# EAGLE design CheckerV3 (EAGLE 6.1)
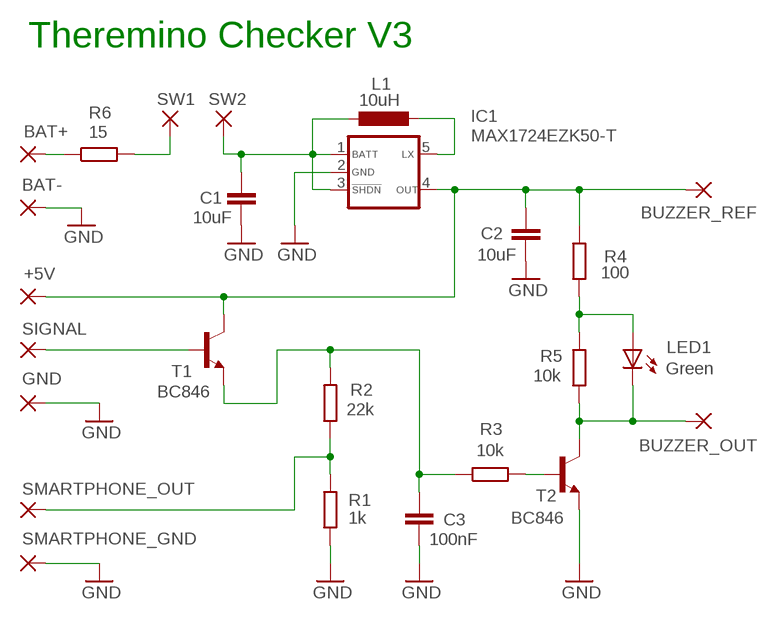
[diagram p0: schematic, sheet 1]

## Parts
+5V  WIREPADSMD1,27-254  [SMD1,27-2,54]
BAT+  WIREPAD2,54/0,9  [2,54/0,9]
BAT-  WIREPAD2,54/0,9  [2,54/0,9]
BUZZER_OUT  WIREPADSMD1,27-254  [SMD1,27-2,54]
BUZZER_REF  WIREPADSMD1,27-254  [SMD1,27-2,54]
C1  10uF  C-EUC0805  [C0805]
C2  10uF  C-EUC0805  [C0805]
C3  100nF  C-EUC0805  [C0805]
GND  WIREPADSMD1,27-254  [SMD1,27-2,54]
IC1  MAX1724EZK50-T  MAX1724SOT23-5-L08  [SOT23-5-L08]
L1  10uH  INDUCTORL1812  [L1812]
LED1  Green  LEDLED3MM-SMD  [LED3MM-SMD]
R1  1k  R-EU_R0805  [R0805]
R2  22k  R-EU_R0805  [R0805]
R3  10k  R-EU_R0805  [R0805]
R4  100  R-EU_R0805  [R0805]
R5  10k  R-EU_R0805  [R0805]
R6  15  R-EU_R0805  [R0805]
SIGNAL  WIREPADSMD1,27-254  [SMD1,27-2,54]
SMARTPHONE_GND  WIREPADSMD1,27-254  [SMD1,27-2,54]
SMARTPHONE_OUT  WIREPADSMD1,27-254  [SMD1,27-2,54]
SW1  WIREPADSMD1,27-254  [SMD1,27-2,54]
SW2  WIREPADSMD1,27-254  [SMD1,27-2,54]
T1  BC846  BC846N  [SOT23]
T2  BC846  BC846N  [SOT23]

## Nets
+BAT: C1.1 IC1.1 IC1.3 L1.1 SW2.1(P)
GND: BAT-.1(P) C1.2 C2.2 C3.2 GND.1(P) IC1.2 R1.1 SMARTPHONE_GND.1(P) T2.2(E)
N$1: LED1.A R4.2 R5.1
N$2: IC1.5 L1.2
N$3: +5V.1(P) BUZZER_REF.1(P) C2.1 IC1.4 R4.1 T1.3(C)
N$4: BUZZER_OUT.1(P) LED1.K(C) R5.2 T2.3(C)
N$5: SIGNAL.1(P) T1.1(B)
N$6: R3.2 T2.1(B)
N$7: R6.2 SW1.1(P)
N$8: C3.1 R2.2 R3.1 T1.2(E)
N$9: R1.2 R2.1 SMARTPHONE_OUT.1(P)
N$10: BAT+.1(P) R6.1

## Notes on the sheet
- Theremino Checker V3

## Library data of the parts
+5V BAT+ BAT- BUZZER_OUT BUZZER_REF GND SIGNAL SMARTPHONE_GND SMARTPHONE_OUT SW1 SW2 = wirepad:WIREPAD: Wire PAD connect wire on PCB
C1-C3 = 00-LIVIO:C-EU: CAPACITOR, European symbol
IC1 = 00-LIVIO:MAX1724: 1.5uA Step-Up DC-DC Converter
L1 = 00-LIVIO:INDUCTOR
LED1 = 00-LIVIO:LED: LEDS
R1-R6 = 00-LIVIO:R-EU_: RESISTOR, European symbol
T1 T2 = 00-LIVIO:BC846

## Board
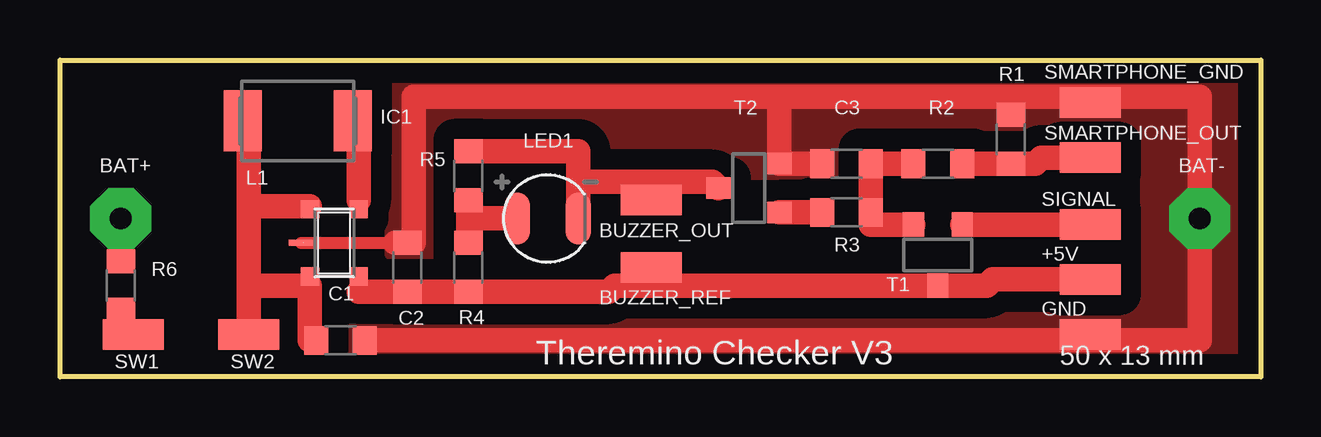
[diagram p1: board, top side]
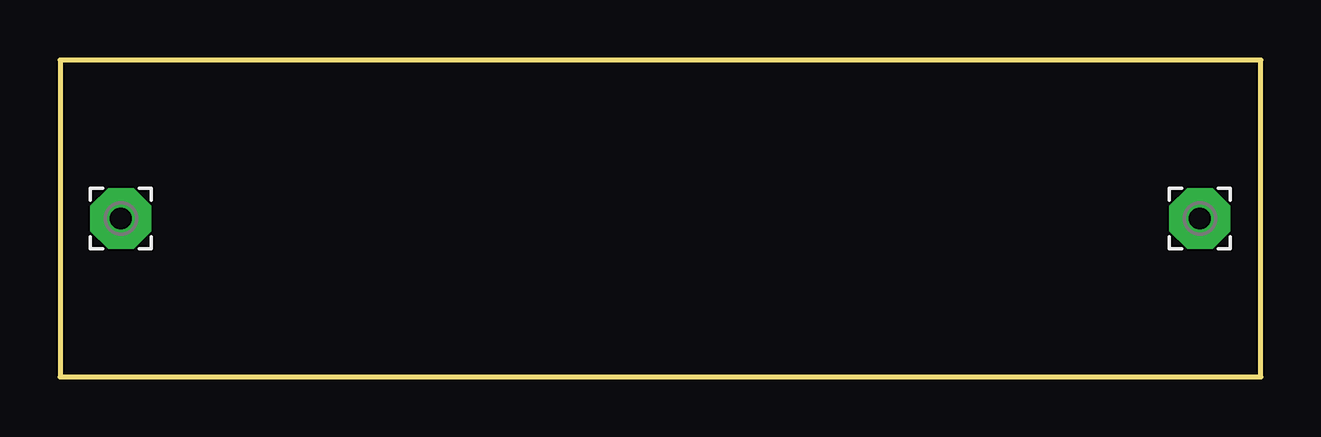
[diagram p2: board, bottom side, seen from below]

Size 50.04 x 13.21 mm. Coordinates in mm from the lower left corner, seen from the top.
Outline: 0,0 0,13.21 50.04,13.21 50.04,0 0,0
Copper layers (1*16): Top 0.035mm / dielectric 1.5mm / Bottom 0.035mm
Design rules: minimum track width 10mil, minimum drill 29mil, track to track 29mil, track to pad 29mil, pad to pad 29mil, via to via 29mil, smd to smd 29mil, copper to edge 29mil, drill to drill 8mil, minimum pad ring 5mil, minimum via ring 8mil, stop-mask expansion 4mil, vias tented up to drill 0mil, thermal gap 44mil

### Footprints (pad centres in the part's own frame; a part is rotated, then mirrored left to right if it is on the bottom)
SMD1,27-2,54 = smd 1.27 x 2.54: 1 0,0
2,54/0,9 = drill 0.914 pad 2.54 octagon: 1 0,0
C0805 = smd 1 x 1.2: 1 -1.016,0; 2 1.016,0
SOT23-5-L08 = smd 0.762 x 0.762: 1 -1.397,-1.016; 3 1.397,-1.016; 4 1.397,1.016; 5 -1.397,1.016 | smd 0.254 x 0.991: 2 0,-1.397
L1812 = smd 1.575 x 2.54: 1 -2.286,0; 2 2.286,0
LED3MM-SMD = smd 1.067 x 2.184: A -1.27,0; K 1.27,0
R0805 = smd 1 x 1.2: 1 -1.016,0; 2 1.016,0
SOT23 = smd 0.889 x 1.016: 1 -1.016,-1.27; 2 1.016,-1.27; 3 0,1.27

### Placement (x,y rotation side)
+5V  42.93,4.06 90 top
BAT+  2.54,6.6 0 bottom
BAT-  47.5,6.6 0 bottom
BUZZER_OUT  24.64,7.37 90 top
BUZZER_REF  24.64,4.57 90 top
C1  11.68,1.52 0 top
C2  14.48,4.57 90 top
C3  32.77,8.89 180 top
GND  42.93,1.78 90 top
IC1  11.43,5.59 270 top
L1  9.91,10.67 0 top
LED1  20.32,6.6 0 top
R1  39.62,9.91 270 top
R2  36.58,8.89 180 top
R3  32.77,6.86 180 top
R4  17.02,4.57 90 top
R5  17.02,8.38 90 top
R6  2.54,3.81 270 top
SIGNAL  42.93,6.35 90 top
SMARTPHONE_GND  42.93,11.43 90 top
SMARTPHONE_OUT  42.93,9.14 90 top
SW1  3.05,1.78 90 top
SW2  7.87,1.78 90 top
T1  36.58,5.08 180 top
T2  28.7,7.87 90 top

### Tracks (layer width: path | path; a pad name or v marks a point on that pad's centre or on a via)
+BAT
  Top 0.61: IC1.3 10.41,3.81 | IC1.1 10.41,7.11 | 7.87,10.67 L1.1
  Top 1.016: 10.41,7.11 7.87,7.11 | L1.1 7.87,10.67 7.87,7.11 | C1.1 10.41,1.52 10.41,3.81 7.87,3.81 | 7.87,3.81 SW2.1 | 7.87,7.11 7.87,3.81
GND
  Top 0.5: IC1.2 13.97,5.59
  Top 0.61: 14.73,5.59 14.73,11.68
  Top 1.016: C3.2 T2.2 29.97,11.68 | 13.97,5.59 C2.2 | C2.2 14.73,5.59 | 43.18,1.52 47.5,1.52 BAT-.1 47.5,11.68 42.93,11.68 | 43.18,1.52 42.93,1.52 GND.1 | 14.73,5.59 14.73,11.68 29.97,11.68 | 29.97,11.68 39.62,11.68 | R1.1 39.62,11.68 | SMARTPHONE_GND.1 42.93,11.68 | C1.2 40.39,1.52 43.18,1.52 | 42.93,11.68 39.62,11.68 | C2.2 14.73,5.59
  pour Top (isolate 0.85, rank 6, no thermals): -1,-1 51.04,-1 51.04,14.21 -1,14.21
N$1
  Top 1.016: LED1.A 17.02,6.6 | 17.02,6.6 R4.2 | R5.1 17.02,6.6
N$2
  Top 0.61: 12.45,7.37 IC1.5
  Top 1.016: L1.2 12.45,10.67 12.45,7.37
N$3
  Top 0.61: IC1.4 12.45,4.06 12.45,3.56
  Top 1.016: 23.11,3.81 22.86,3.56 R4.1 C2.1 12.45,3.56 | 23.11,3.81 24.64,3.81 | 24.64,3.81 T1.3 38.61,3.81 38.86,4.06 40.64,4.06 +5V.1 | BUZZER_REF.1 24.64,3.81 | 24.64,3.81 23.11,3.81
N$4
  Top 1.016: T2.3 27.18,8.13 24.64,8.13 | 24.64,8.13 21.59,8.13 | 21.59,8.13 LED1.K | BUZZER_OUT.1 24.64,8.13 | R5.2 21.59,9.4 21.59,8.13
N$5
  Top 1.016: SIGNAL.1 40.39,6.35 40.13,6.35 T1.1
N$6
  Top 1.016: R3.2 T2.1
N$7
  Top 1.016: R6.2 2.54,1.78 SW1.1
N$8
  Top 1.016: R2.2 C3.1 R3.1 33.78,6.35 T1.2
N$9
  Top 1.016: R2.1 R1.2 40.64,8.89 40.89,9.14 SMARTPHONE_OUT.1
N$10
  Top 1.016: R6.1 BAT+.1

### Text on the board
tNames: Theremino Checker V3 | 50 x 13 mm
